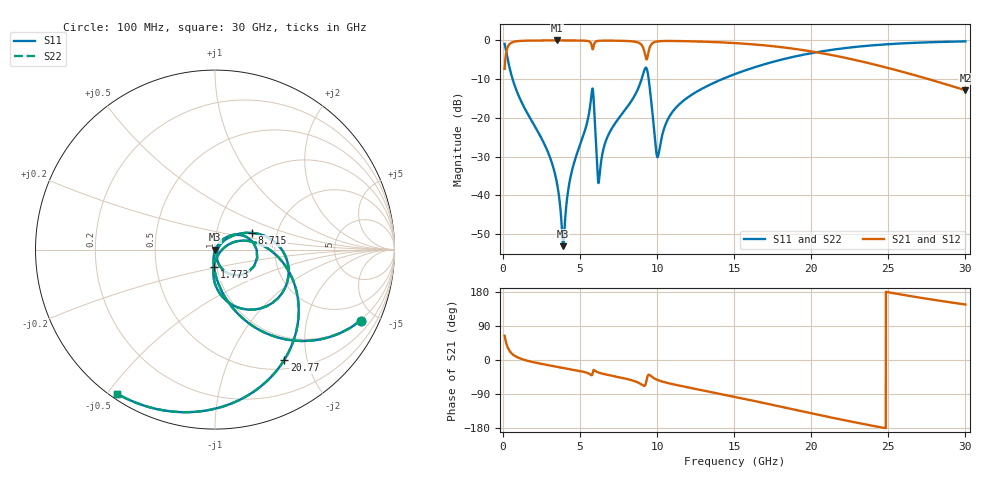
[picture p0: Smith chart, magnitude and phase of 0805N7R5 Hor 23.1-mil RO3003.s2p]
# GHz S MA R 50
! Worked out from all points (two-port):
!   3201 points, 100 MHz to 30 GHz, reference 50 ohm
!   highest |S21| = -0.02 dB at 3.51 GHz (marker M1); lowest = -12.9 dB at 30 GHz (marker M2)
!   |S21| within 3 dB of the highest: 209.9 MHz to 9.176 GHz (8.967 GHz wide, 191 % of centre); 9.437 GHz to 20.27 GHz (10.83 GHz wide, 72.9 % of centre)
!   lowest |S11| = -53.1 dB at 3.903 GHz (marker M3), VSWR 1.00, Z = 50.2 - j0.0827 ohm
!   |S11| at or under -10 dB: 618.6 MHz to 8.989 GHz (8.37 GHz wide, 174 % of centre); 9.449 GHz to 14.22 GHz (4.774 GHz wide, 40.3 % of centre)
!   |S22| runs from -53.1 to -0.3 dB; largest |S21 - S12| = 0
!   S11 on the Smith chart (normalised r, x): 100 MHz: 0.96, -4.13; 1.773 GHz: 0.97, -0.19; 8.715 GHz: 1.49, +0.29; 20.77 GHz: 0.63, -1.63; 30 GHz: 0.02, -0.53
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0.1  0.9031 -25.9  0.4291 64.0  0.4291 64.0  0.9031 -25.9
0.5671875  0.3427 -72.9  0.9387 17.0  0.9387 17.0  0.3427 -72.9
1.772531  0.09789 -93.1  0.9938 -3.9  0.9938 -3.9  0.09789 -93.1
3.510469  0.01393 -99.7  0.9978 -18.0  0.9978 -18.0  0.01393 -99.7
3.902906  0.002214 -21.8  0.9976 -20.9  0.9976 -20.9  0.002214 -21.8
4.379437  0.01734 57.1  0.9971 -24.4  0.9971 -24.4  0.01734 57.1
5.089563  0.05071 55.0  0.9941 -30.0  0.9941 -30.0  0.05071 55.0
5.781  0.2325 -0.6  0.8072 -39.0  0.8072 -39.0  0.2325 -0.6
5.902469  0.1407 -63.9  0.8845 -26.4  0.8845 -26.4  0.1407 -63.9
6.117375  0.02118 -59.0  0.9809 -31.9  0.9809 -31.9  0.02118 -59.0
6.248188  0.01712 14.6  0.9883 -33.9  0.9883 -33.9  0.01712 14.6
6.836844  0.0606 45.2  0.9924 -39.6  0.9924 -39.6  0.0606 45.2
8.714937  0.2273 24.2  0.9458 -58.7  0.9458 -58.7  0.2273 24.2
9.331625  0.4274 -47.5  0.5724 -49.6  0.5724 -49.6  0.4274 -47.5
9.602594  0.1723 -91.5  0.878 -42.6  0.878 -42.6  0.1723 -91.5
10.06978  0.03267 -18.9  0.9725 -53.4  0.9725 -53.4  0.03267 -18.9
11.32184  0.1425 19.8  0.9805 -66.6  0.9805 -66.6  0.1425 19.8
15.05  0.3678 -8.5  0.9225 -97.4  0.9225 -97.4  0.3678 -8.5
20.03956  0.6858 -51.6  0.7188 -140.9  0.7188 -140.9  0.6858 -51.6
20.76837  0.7261 -57.9  0.6784 -147.3  0.6784 -147.3  0.7261 -57.9
25.01978  0.8935 -91.9  0.4387 178.6  0.4387 178.6  0.8935 -91.9
30  0.9707 -124.1  0.2273 146.5  0.2273 146.5  0.9707 -124.1
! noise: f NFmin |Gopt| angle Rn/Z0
0.1  0.0007383  0.9167  0.9987  0.001956
3.417  0.006235  0.7006  18.37  0.003977
6.743  0.01471  0.7473  35.54  0.01064
10.06  0.03908  0.8532  52.29  0.04583
13.39  0.02267  0.7  67.15  0.01041
16.7  0.02722  0.6984  81.17  0.01041
20.03  0.03444  0.7209  94.55  0.0116
23.35  0.04473  0.7555  107.5  0.01341
26.67  0.06004  0.7983  120.3  0.01587
30  0.08427  0.8452  133.1  0.01897
